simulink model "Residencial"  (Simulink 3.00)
settings: Solver=ode45  StartTime=0.0  StopTime=250  FixedStep=0.1  RelTol=1e-3  AbsTol=1e-3

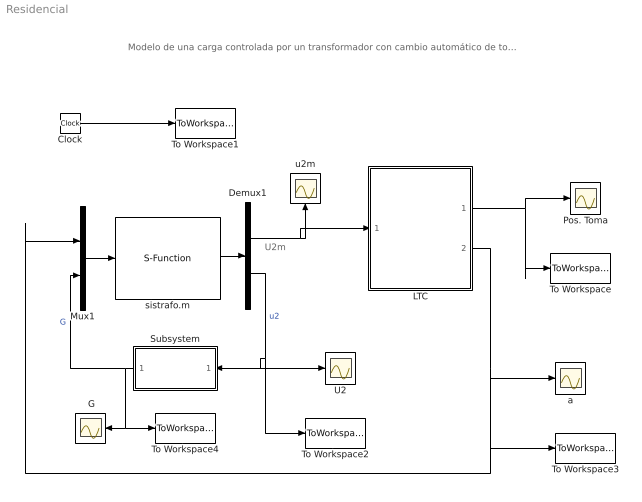
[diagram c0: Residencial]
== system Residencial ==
  note: U2m
  note: Modelo de una carga controlada por un transformador con cambio automático de tomas
  " G" : Scope
  Clock : Clock
  Demux1 : Demux  Outputs=2
  LTC : Subsystem  mask{incrtoma=0.00625, tmax=16, tmin=-16, tinic=-4, Td=30, Tm=5, DB=0.00833, Uref=1.0}
      mask prompts: incrtoma "Pasos discretos de la toma"; tmax "Posición máxima de la toma, tmax."; tmin "Posición mínima de la toma, tmin."; tinic "Posición inicial de la toma, tinic."; Td "Tiempo de retardo de la actuación, Td [ sg. ]"; Tm "Tiempo del mecanismo de actuación, Tm  [ sg. ]"; DB "Zona muerta,  DB  [ p.u. ]"; Uref "Tensión de Referencia,  Uref  [ p. u. ]"
  Mux1 : Mux  Inputs=2
  Pos. Toma : Scope
  Subsystem : Subsystem  Orientation=left  mask{Pter=1.5, Go=1.5, Kl=4, Tter=60}
      mask prompts: Pter "Potencia Activa termostática [pu.]"; Go "Valor inicial de la Conductancia Termostática Go [ pu.]"; Kl "Máximo número de veces de Go"; Tter "Retardo termostático [seg.]"
  To Workspace : ToWorkspace  VariableName=Pos  SampleTime=-1  SaveFormat=Matrix
  To Workspace1 : ToWorkspace  VariableName=t  SampleTime=-1  SaveFormat=Matrix
  To Workspace2 : ToWorkspace  VariableName=U2  SampleTime=-1  SaveFormat=Matrix
  To Workspace3 : ToWorkspace  VariableName=a  SampleTime=-1  SaveFormat=Matrix
  To Workspace4 : ToWorkspace  VariableName=G  SampleTime=-1  SaveFormat=Matrix
  U2 : Scope
  a : Scope
  sistrafo.m : S-Function  FunctionName=sistrafo  Parameters=U1,gU1,Rtrafo,Xtrafo,Rc,Xc,Kld,P2t,Q2t,Kg,Rload,Rsis,Xsis  PortCounts=[]  SFunctionModules=''  mask{U1=1.0788, gU1=5.0972, Rsis=0.01, Xsis=0.0636057, Rtrafo=0.00, Xtrafo=0.01, Rc=0.0, Xc=0.0, Kld=0, P2t=0, Kg=1, Rload=0.666666, Q2t=0.5}
      mask prompts: U1 "Módulo de la tensión del primario [ pu. ]"; gU1 "Angulo de la Tensión del Primario [ ° ]"; Rsis "Resistencia del Sistema Equivalente [ pu.]"; Xsis "Reactancia del Sistema Equivalente [ pu. ]"; Rtrafo "Resistencia del Trafo  [ pu. ]"; Xtrafo "Reactancia del Trafo [pu.]"; Rc "Resistencia de Compensación Line Drop  [ pu.]"; Xc "Reactancia de compensación Line Drop  [ pu. ]"; Kld "Factor de compensación Line Drop"; P2t "Potencia Activa de la Carga constante  [ pu. ]"; Kg "Modelo carga termostática (1: si   0: no)"; Rload "Resistencia de carga constante [pu.]"; Q2t "Potencia Reactiva de la carga constante [ pu. ]"
  u2m : Scope
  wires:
  Mux1/1 -> sistrafo.m/1
  sistrafo.m/1 -> Demux1/1
  Subsystem/1(G) -> Mux1/2, " G"/1, To Workspace4/1  "G"
  LTC/1(Pos. Toma) -> Pos. Toma/1, To Workspace/1
  Demux1/2 -> Subsystem/1(U2), U2/1, To Workspace2/1  "u2"
  Demux1/1 -> LTC/1(U2m), u2m/1
  Clock/1 -> To Workspace1/1
  LTC/2(a) -> a/1, Mux1/1, To Workspace3/1

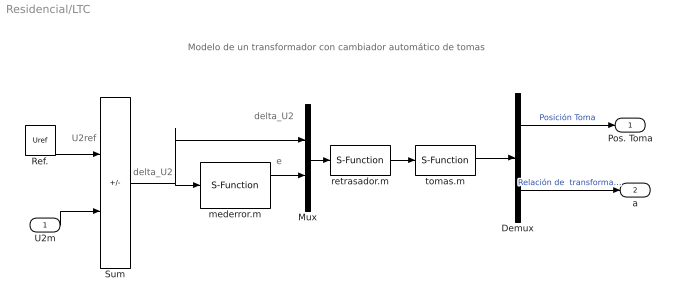
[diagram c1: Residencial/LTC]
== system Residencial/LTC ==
  note: U2ref
  note: delta_U2
  note: e
  note: delta_U2
  note: Modelo de un transformador con cambiador automático de tomas
  U2m : Inport  Port=1  PortWidth=-1  SampleTime=-1  DataType=auto
  Demux : Demux  Outputs=2
  Mux : Mux  Inputs=2
  Ref. : Constant  Value=Uref
  Sum : Sum  Inputs=+-  SaturateOnIntegerOverflow=on
  mederror.m : S-Function  FunctionName=Mederror  Parameters=DB  PortCounts=[]  SFunctionModules=''  mask{DB=DB}
      mask prompts: DB "Variación de tensión que detecta"
  retrasador.m : S-Function  FunctionName=retrasador  Parameters=DB,Tdo  PortCounts=[]  SFunctionModules=''  mask{Tdo=Td, DB=DB}
      mask prompts: Tdo "Retraso Inicial [seg.]"; DB "Variación de tensión que detecta"
  tomas.m : S-Function  FunctionName=tomas  Parameters=incrtoma,tinic,tmin,tmax  PortCounts=[]  SFunctionModules=''  mask{incrtoma=incrtoma, tmax=tmax, tmin=tmin, tinic=tinic}
      mask prompts: incrtoma "Paso de incremento de la toma"; tmax "Posición Máxima de la toma"; tmin "Posición Mínima de la toma"; tinic "Posición Inicial de la toma"
  Pos. Toma : Outport  Port=1
  a : Outport  Port=2
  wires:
  Mux/1 -> retrasador.m/1
  tomas.m/1 -> Demux/1
  retrasador.m/1 -> tomas.m/1
  mederror.m/1 -> Mux/2
  Demux/1 -> Pos. Toma/1  "Posición Toma"
  Demux/2 -> a/1  "Relación de  transformación 'a'"
  Ref./1 -> Sum/1
  U2m/1 -> Sum/2
  Sum/1 -> mederror.m/1, Mux/1

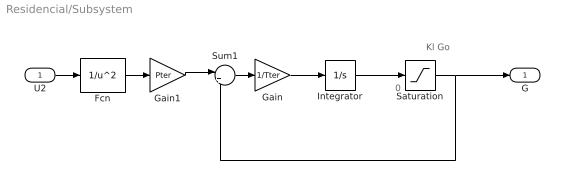
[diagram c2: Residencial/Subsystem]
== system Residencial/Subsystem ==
  note: Kl Go
  note: 0
  U2 : Inport  Port=1  PortWidth=-1  SampleTime=-1  DataType=auto
  Fcn : Fcn  Expr=1/u^2
  Gain : Gain  Gain=1/Tter  SaturateOnIntegerOverflow=on
  Gain1 : Gain  Gain=Pter  SaturateOnIntegerOverflow=on
  Integrator : Integrator  ExternalReset=none  InitialConditionSource=internal  InitialCondition=Go  LimitOutput=off  UpperSaturationLimit=inf  LowerSaturationLimit=-inf  ShowSaturationPort=off  ShowStatePort=off  AbsoluteTolerance=auto
  Saturation : Saturate  UpperLimit=Kl*Go  LowerLimit=0
  Sum1 : Sum  Inputs=|+-  SaturateOnIntegerOverflow=on
  G : Outport  Port=1
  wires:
  Gain1/1 -> Sum1/1
  Sum1/1 -> Gain/1
  Gain/1 -> Integrator/1
  Integrator/1 -> Saturation/1
  Saturation/1 -> Sum1/2, G/1
  Fcn/1 -> Gain1/1
  U2/1 -> Fcn/1
